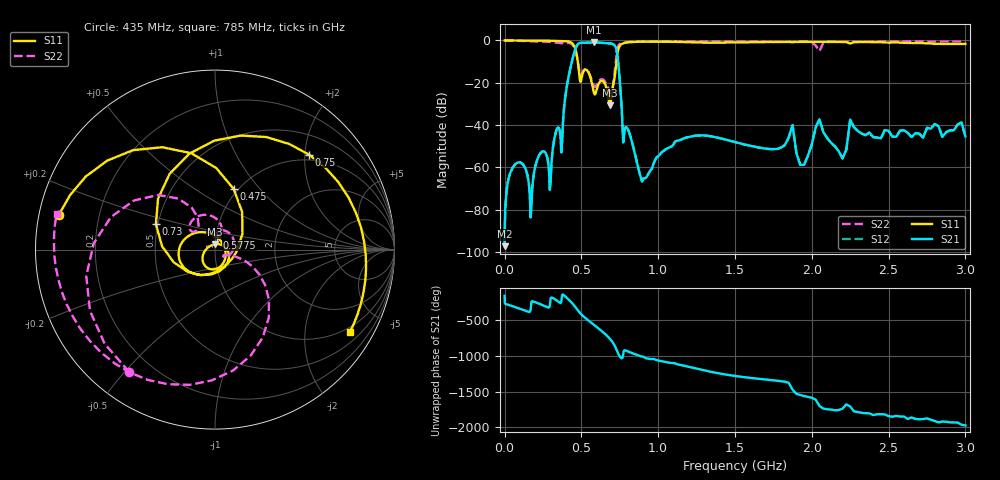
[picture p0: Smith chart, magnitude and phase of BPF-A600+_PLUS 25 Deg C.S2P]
! Mini-Circuits
! S2P DATA File Format
! Type: BAND PASS FILTER
! Model:BPF-A600+
! All S Parameters are in dB deg format
! TEST CONDITIONS: INPUT POWER = 0 dBm @ Temperature = + 25 deg C
! 401 Frequency points
# MHz S DB R 50
!FREQMAG(S11)PHS(S11)MAG(S21)PHS(S21)MAG(S12)PHS(S12)MAG(S22)PHS(S22)
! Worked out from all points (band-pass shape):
!   401 points, 500 kHz to 3 GHz, reference 50 ohm
!   highest |S21| = -0.93 dB at 580 MHz (marker M1); lowest = -97.2 dB at 500 kHz (marker M2)
!   |S21| within 3 dB of the highest: 461.6 MHz to 727 MHz (265.4 MHz wide, 44.6 % of centre)
!   lowest |S11| = -30.7 dB at 687.5 MHz (marker M3), VSWR 1.06, Z = 49.7 + j2.9 ohm
!   |S11| at or under -10 dB: 476.8 MHz to 728.4 MHz (251.6 MHz wide, 41.8 % of centre)
!   |S22| runs from -24.8 to 0.0 dB; largest |S21 - S12| = 0.0011
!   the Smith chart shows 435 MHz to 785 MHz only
!   S11 on the Smith chart (normalised r, x): 435 MHz: 0.06, +0.11; 475 MHz: 0.95, +0.74; 577.5 MHz: 1.01, +0.14; 730 MHz: 0.49, +0.16; 750 MHz: 0.88, +2.09; 785 MHz: 0.82, -3.36
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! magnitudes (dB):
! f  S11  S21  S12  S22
! 500 kHz  0.0  -97.2  -96.8  0.0
! 75 MHz  0.0  -58.1  -58.1  -0.1
! 170 MHz  0.0  -83.6  -84.6  -0.4
! 235 MHz  -0.1  -53.1  -53.2  -0.5
! 295 MHz  -0.1  -70.6  -70.2  -0.7
! 375 MHz  -0.2  -47.4  -47.4  -1.3
! 435 MHz  -1.0  -11.0  -11.0  -1.6
! 475 MHz  -9.0  -2.0  -2.0  -9.1
! 502.5 MHz  -17.4  -1.1  -1.1  -15.8
! 577.5 MHz  -23.3  -0.9  -0.9  -20.8
! 580 MHz  -24.1  -0.9  -0.9  -21.2
! 687.5 MHz  -30.7  -1.4  -1.4  -24.6
! 730 MHz  -8.9  -4.9  -4.9  -6.3
! 750 MHz  -2.6  -18.7  -18.7  -1.6
! 772.5 MHz  -1.4  -48.1  -48.1  -1.0
! 785 MHz  -1.1  -41.4  -41.4  -0.9
! 892.5 MHz  -0.6  -66.1  -65.8  -0.5
! 1.01 GHz  -0.6  -54.0  -53.9  -0.5
! 1.51 GHz  -0.9  -48.2  -48.2  -0.5
! 2.025 GHz  -0.7  -41.2  -41.2  -2.3
! 2.525 GHz  -1.0  -45.5  -45.4  -0.5
! 3 GHz  -1.6  -45.3  -45.3  -0.5
